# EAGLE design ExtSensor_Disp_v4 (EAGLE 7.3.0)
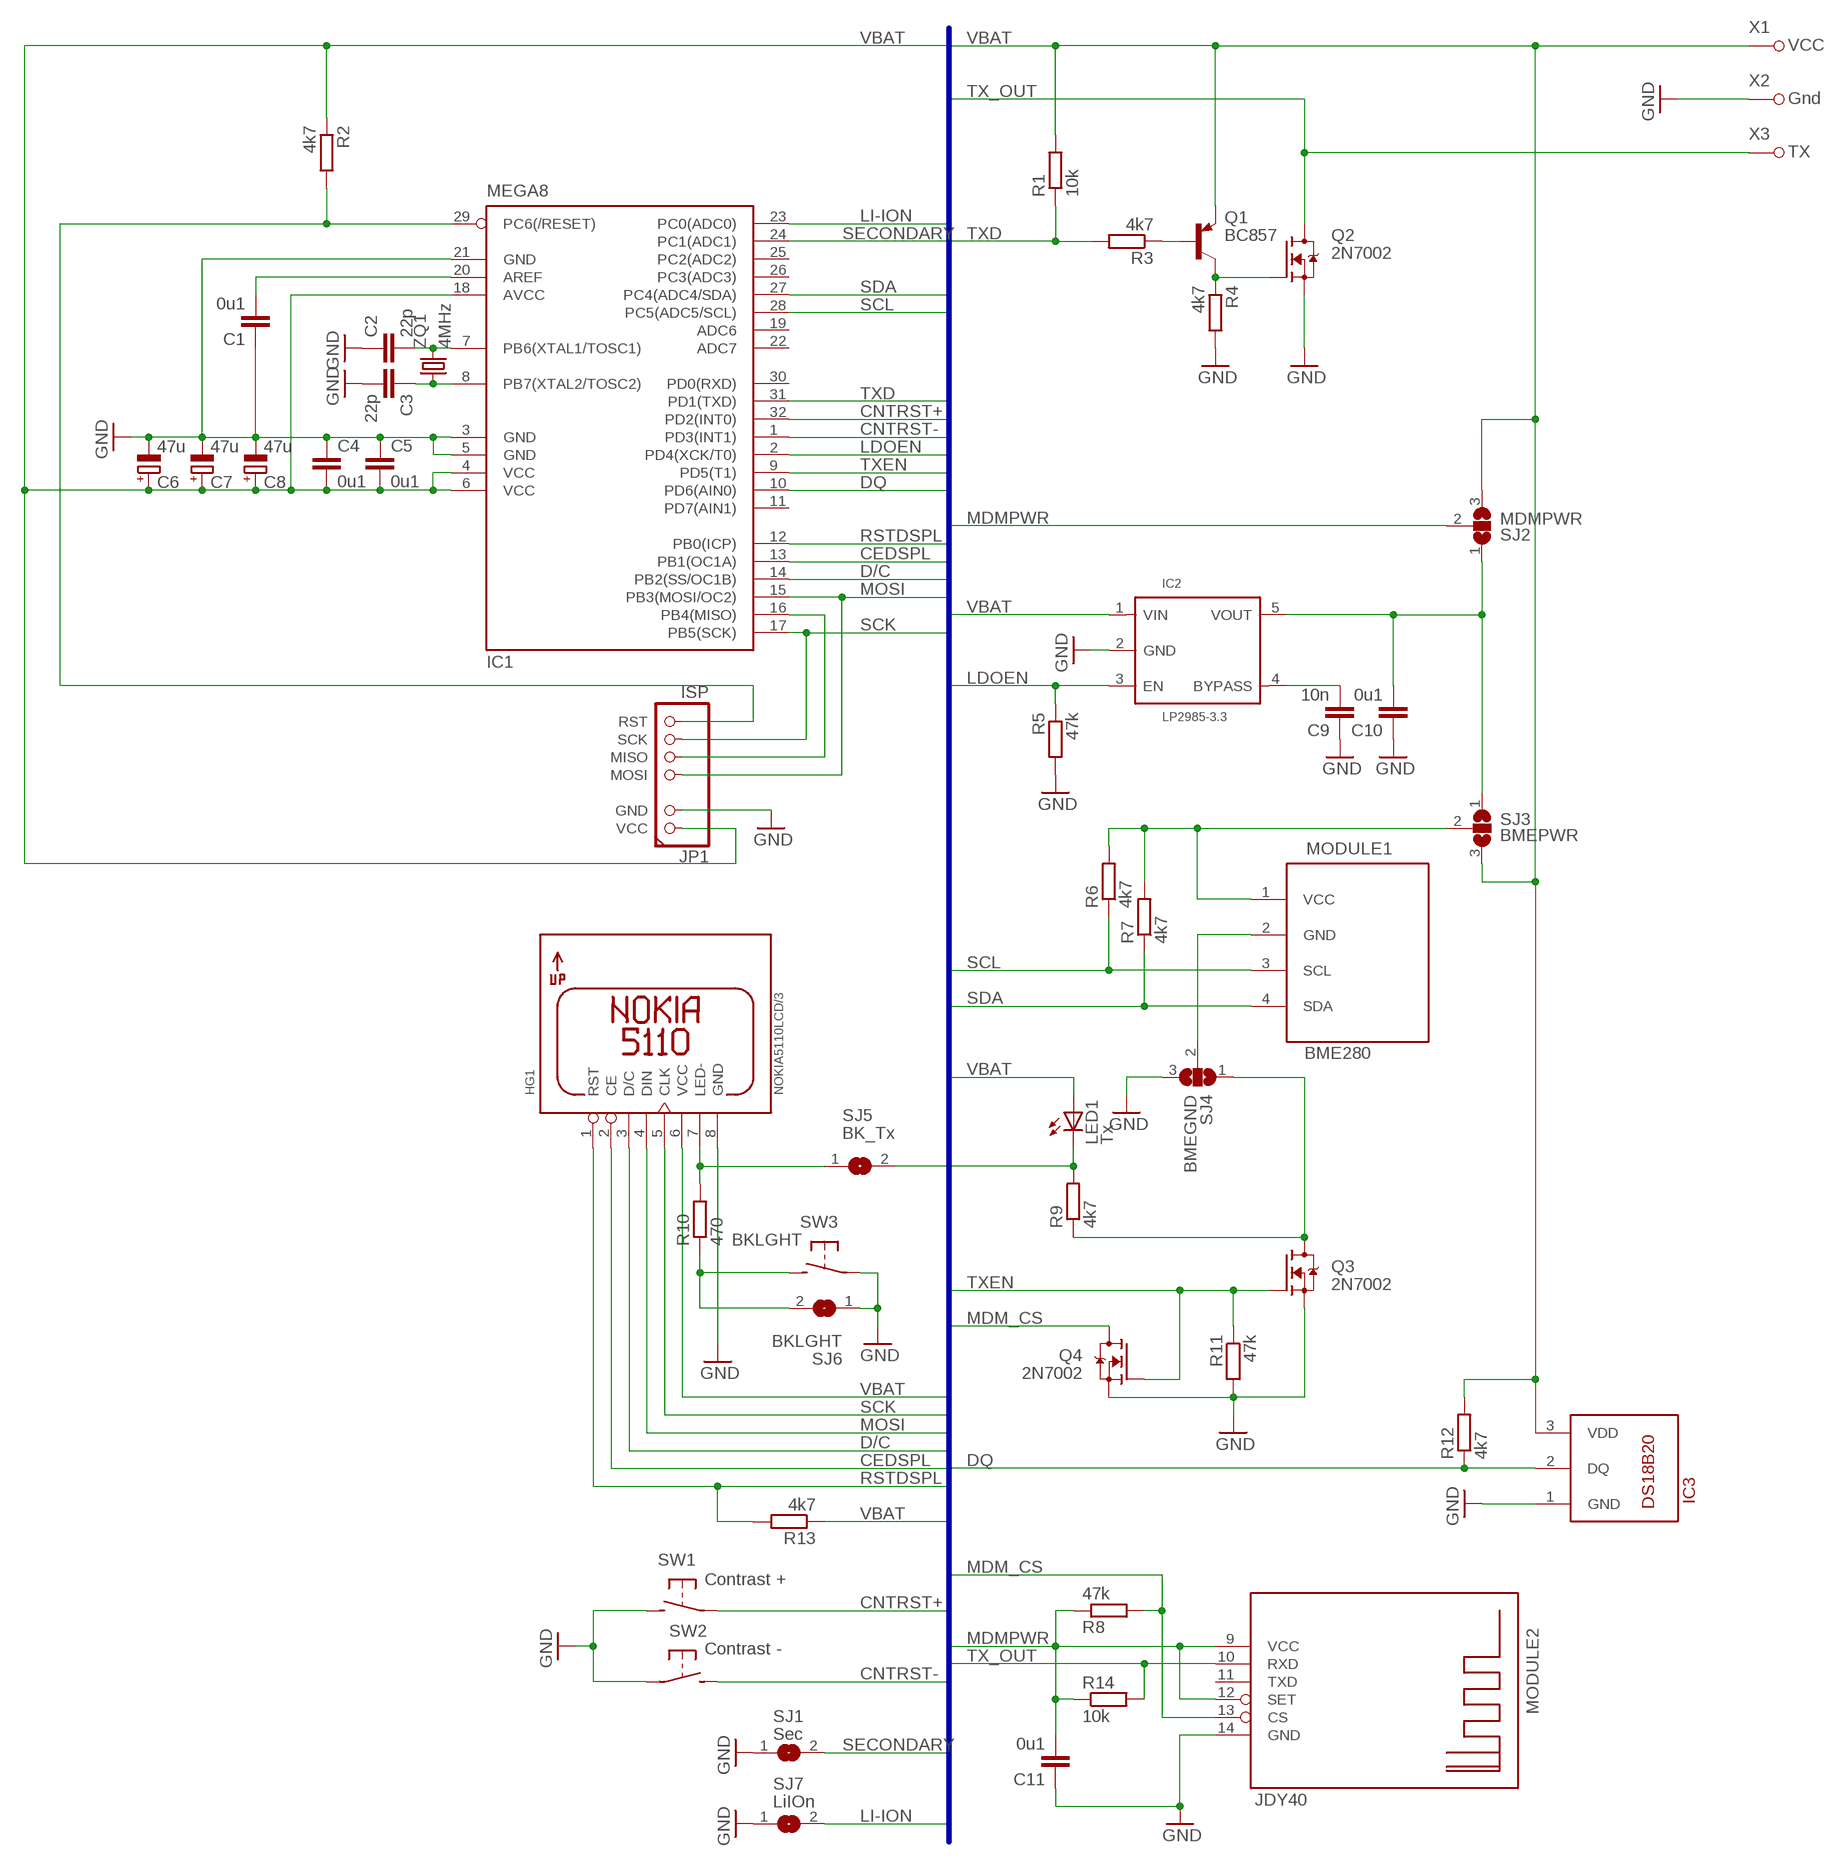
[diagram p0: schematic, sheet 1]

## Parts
C1  0u1  C-EUC0805T  [C0805T]
C2  22p  C-EUC0805T  [C0805T]
C3  22p  C-EUC0805T  [C0805T]
C4  0u1  C-EUC0805T  [C0805T]
C5  0u1  C-EUC0805T  [C0805T]
C6  47u  CPOL-EUE2.5-6  [E2,5-6]
C7  47u  CPOL-EUSMCB  [SMC_B]
C8  47u  CPOL-EUSMCB  [SMC_B]
C9  10n  C-EUC0805T  [C0805T]
C10  0u1  C-EUC0805T  [C0805T]
C11  0u1  C-EUC0805T  [C0805T]
HG1  NOKIA5110LCD/3  [NOKIA5110LCD_V3_NOSILK]
IC1  MEGA8  MEGA8-AI  [TQFP32-08]
IC2  LP2985-3.3  LP2985-XX  [SOT23-5]
IC3  DS18B20  DS18B20/-BH  [TO92-/BIG_HOLES]
JP1  ISP  CONN1X7(2+4)_ISP+/P/NI  [1X07_ISP+POINTS_NO_INF]
LED1  Tx  LED3MM  [LED3MM]
MODULE1  BME280  BM(P|E)280_I2C/4  [BM(P|E)280_I2C_5V]
MODULE2  JDY40  JDY40_NO_GPIO/SMD  [JDY40_NG_SMD]
Q1  BC857  BC857THIN  [SOT23_THIN]
Q2  2N7002  2N7002/THIN  [SOT23_THIN]
Q3  2N7002  2N7002/THIN  [SOT23_THIN]
Q4  2N7002  2N7002/THIN  [SOT23_THIN]
R1  10k  R-EU_R0805T  [R0805T]
R2  4k7  R-EU_R0805T  [R0805T]
R3  4k7  R-EU_R0805T  [R0805T]
R4  4k7  R-EU_R0805T  [R0805T]
R5  47k  R-EU_R0805T  [R0805T]
R6  4k7  R-EU_R0805T  [R0805T]
R7  4k7  R-EU_R0805T  [R0805T]
R8  47k  R-EU_R0805T  [R0805T]
R9  4k7  R-EU_R0805T  [R0805T]
R10  470  R-EU_R0805T  [R0805T]
R11  47k  R-EU_R0805T  [R0805T]
R12  4k7  R-EU_R0805T  [R0805T]
R13  4k7  R-EU_R0805T  [R0805T]
R14  10k  R-EU_R0805T  [R0805T]
SJ1  Sec  SJ  [SJ]
SJ2  MDMPWR  SJ2W  [SJ_2]
SJ3  BMEPWR  SJ2W  [SJ_2]
SJ4  BMEGND  SJ2W  [SJ_2]
SJ5  BK_Tx  SJ  [SJ]
SJ6  BKLGHT  SJ  [SJ]
SJ7  LiIOn  SJ  [SJ]
SW1  Contrast +  TACT_BUTTON  [G72]
SW2  Contrast -  TACT_BUTTON  [G72]
SW3  BKLGHT  TACT_BUTTON  [G72]
X1  VCC  SIMPLE_WIRED_HOLE/1.0MM  [SIMPLE_WIRED_HOLE_1.0]
X2  Gnd  SIMPLE_WIRED_HOLE/1.0MM  [SIMPLE_WIRED_HOLE_1.0]
X3  TX  SIMPLE_WIRED_HOLE/1.0MM  [SIMPLE_WIRED_HOLE_1.0]
ZQ1  4MHz  CRYSTAL_AL/TH  [HC49/S]

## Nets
BMEGND: MODULE1.2(GND) SJ4.2
BMEPWR: MODULE1.1(VCC) R6.2 R7.2 SJ3.2
CEDSPL: HG1.2(CE) IC1.13(PB1(OC1A))
CNTRST+: IC1.32(PD2(INT0)) SW1.S1(P)
CNTRST-: IC1.1(PD3(INT1)) SW2.S2(S)
D/C: HG1.3(D/C) IC1.14(PB2(SS/OC1B))
DQ: IC1.10(PD6(AIN0)) IC3.2(DQ) R12.1
GND: C1.1 C2.1 C3.2 C4.1 C5.1 C6.- C7.- C8.- C9.1 C10.1 C11.1 HG1.8(GND) IC1.3(GND) IC1.5(GND) IC1.21(GND) IC2.2(GND) IC3.1(GND) JP1.GND MODULE2.14(GND) Q2.2(S) Q3.2(S) Q4.2(S) R4.2 R5.2 R11.2 SJ1.1 SJ4.3 SJ6.1 SJ7.1 SW1.S2(S) SW2.S1(P) SW3.S1(P) X2.P$1
LDO_OUT: C10.2 IC2.5(VOUT) SJ2.1 SJ3.1
LDOEN: IC1.2(PD4(XCK/T0)) IC2.3(EN) R5.1
LI-ION: IC1.23(PC0(ADC0)) SJ7.2
MDM_CS: MODULE2.13(CS) Q4.3(D) R8.2
MDMPWR: C11.2 MODULE2.9(VCC) MODULE2.12(SET) R8.1 R14.1 SJ2.2
MISO: IC1.16(PB4(MISO)) JP1.MISO
MOSI: HG1.4(DIN) IC1.15(PB3(MOSI/OC2)) JP1.MOSI
N$1: C3.1 IC1.8(PB7(XTAL2/TOSC2)) ZQ1.1
N$2: Q1.3(C) Q2.1(G) R4.1
N$3: C2.2 IC1.7(PB6(XTAL1/TOSC1)) ZQ1.2
N$4: C9.2 IC2.4(BYPASS)
N$5: HG1.7(LED-) R10.2 SJ5.1
N$7: LED1.K(C) R9.2 SJ5.2
N$9: R10.1 SJ6.2 SW3.S2(S)
N$10: C1.2 IC1.20(AREF)
N$12: Q1.1(B) R3.1
N$16: Q3.3(D) R9.1 SJ4.1
RST: IC1.29(PC6(/RESET)) JP1.RST R2.2
RSTDSPL: HG1.1(RST) IC1.12(PB0(ICP)) R13.2
SCK: HG1.5(CLK) IC1.17(PB5(SCK)) JP1.SCK
SCL: IC1.28(PC5(ADC5/SCL)) MODULE1.3(SCL) R6.1
SDA: IC1.27(PC4(ADC4/SDA)) MODULE1.4(SDA) R7.1
SECONDARY: IC1.24(PC1(ADC1)) SJ1.2
TX_OUT: MODULE2.10(RXD) Q2.3(D) R14.2 X3.P$1
TXD: IC1.31(PD1(TXD)) R1.1 R3.2
TXEN: IC1.9(PD5(T1)) Q3.1(G) Q4.1(G) R11.1
VBAT: C4.2 C5.2 C6.+ C7.+ C8.+ HG1.6(VCC) IC1.4(VCC) IC1.6(VCC) IC1.18(AVCC) IC2.1(VIN) IC3.3(VDD) JP1.+5V(VCC) LED1.A Q1.2(E) R1.2 R2.1 R12.2 R13.1 SJ2.3 SJ3.3 X1.P$1
Unconnected: IC1.11(PD7(AIN1)) IC1.19(ADC6) IC1.22(ADC7) IC1.25(PC2(ADC2)) IC1.26(PC3(ADC3)) IC1.30(PD0(RXD)) MODULE2.11(TXD)

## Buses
VBAT,TXD,SCL,SDA,DQ,MOSI,SCK,D/C,CEDSPL,RSTDSPL,LDOEN,CNTRST-,CNTRST+,TXEN,MDM_CS,MDMPWR,TX_OUT,LI-ION,SECONDARY

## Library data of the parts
C1-C5 C9-C11 = rcl:C-EU: CAPACITOR, European symbol
C6-C8 = rcl:CPOL-EU: POLARIZED CAPACITOR, European symbol
HG1 = lcd-AL:NOKIA5110LCD/3
IC1 = atmel:MEGA8: MICROCONTROLLER 8 Kbytes FLASH, 1 kbytes SRAM, 512 bytes EEPROM, USART, 6-channel 10 bit ADC, 2-channel 8 bit ADC Pin compatible with Atmega48, ATMega88, ATMega168 Source: avr.lbr; MPN: ATMEGA8-16AU; OC_FARNELL: 9171371; OC_NEWARK: 73M8863
IC2 = v-reg-AL:LP2985-XX: Texas Instruments LP2985 150-mA Low-noise Low-dropout Regulator With Shutdown
IC3 = misc-active-AL:DS18B20
JP1 = pinhead-AL:CONN1X7(2+4)_ISP+: PIN HEADER
LED1 = led-AL:LED
MODULE1 = modules-external-AL:BM(P|E)280_I2C
MODULE2 = modules-external-AL:JDY40_NO_GPIO
Q1 = transistor-pnp-AL:BC857*: PNP Transistror
Q2-Q4 = transistor-fet-drv-AL:2N7002: Small signal N-Channel MOSFET transistor
R1-R14 = rcl:R-EU_: RESISTOR, European symbol
SJ1 SJ5-SJ7 = jumper:SJ: SMD solder JUMPER
SJ2-SJ4 = jumper:SJ2W: SMD solder JUMPER
SW1-SW3 = switch-misc-AL:TACT_BUTTON
X1-X3 = connectors-AL:SIMPLE_WIRED_HOLE
ZQ1 = crystal:CRYSTAL_AL

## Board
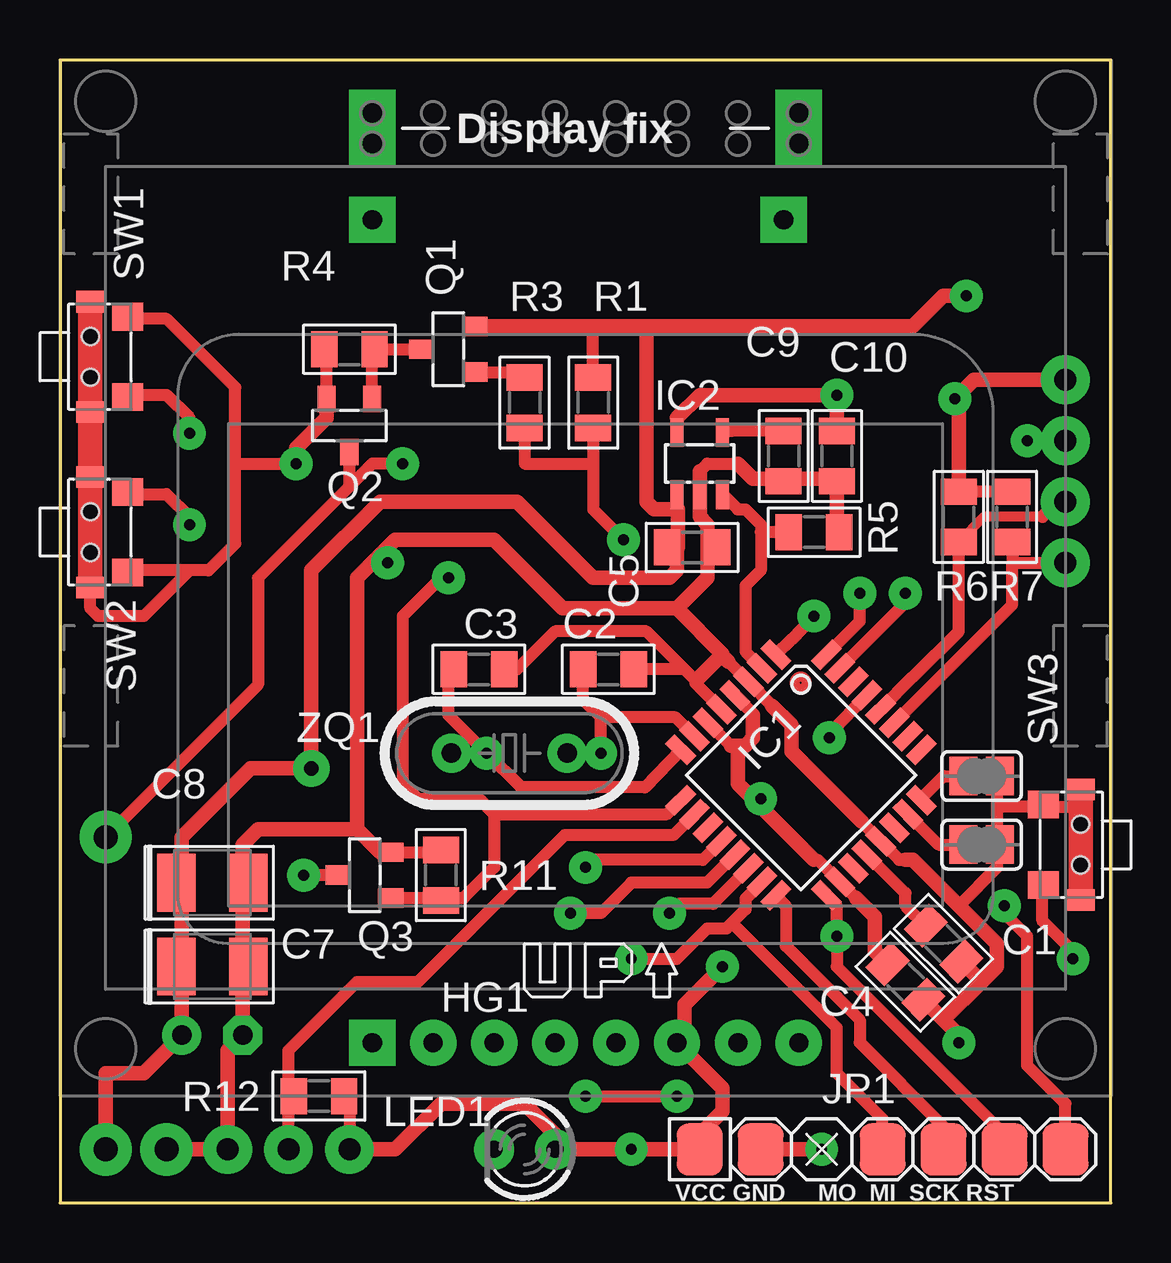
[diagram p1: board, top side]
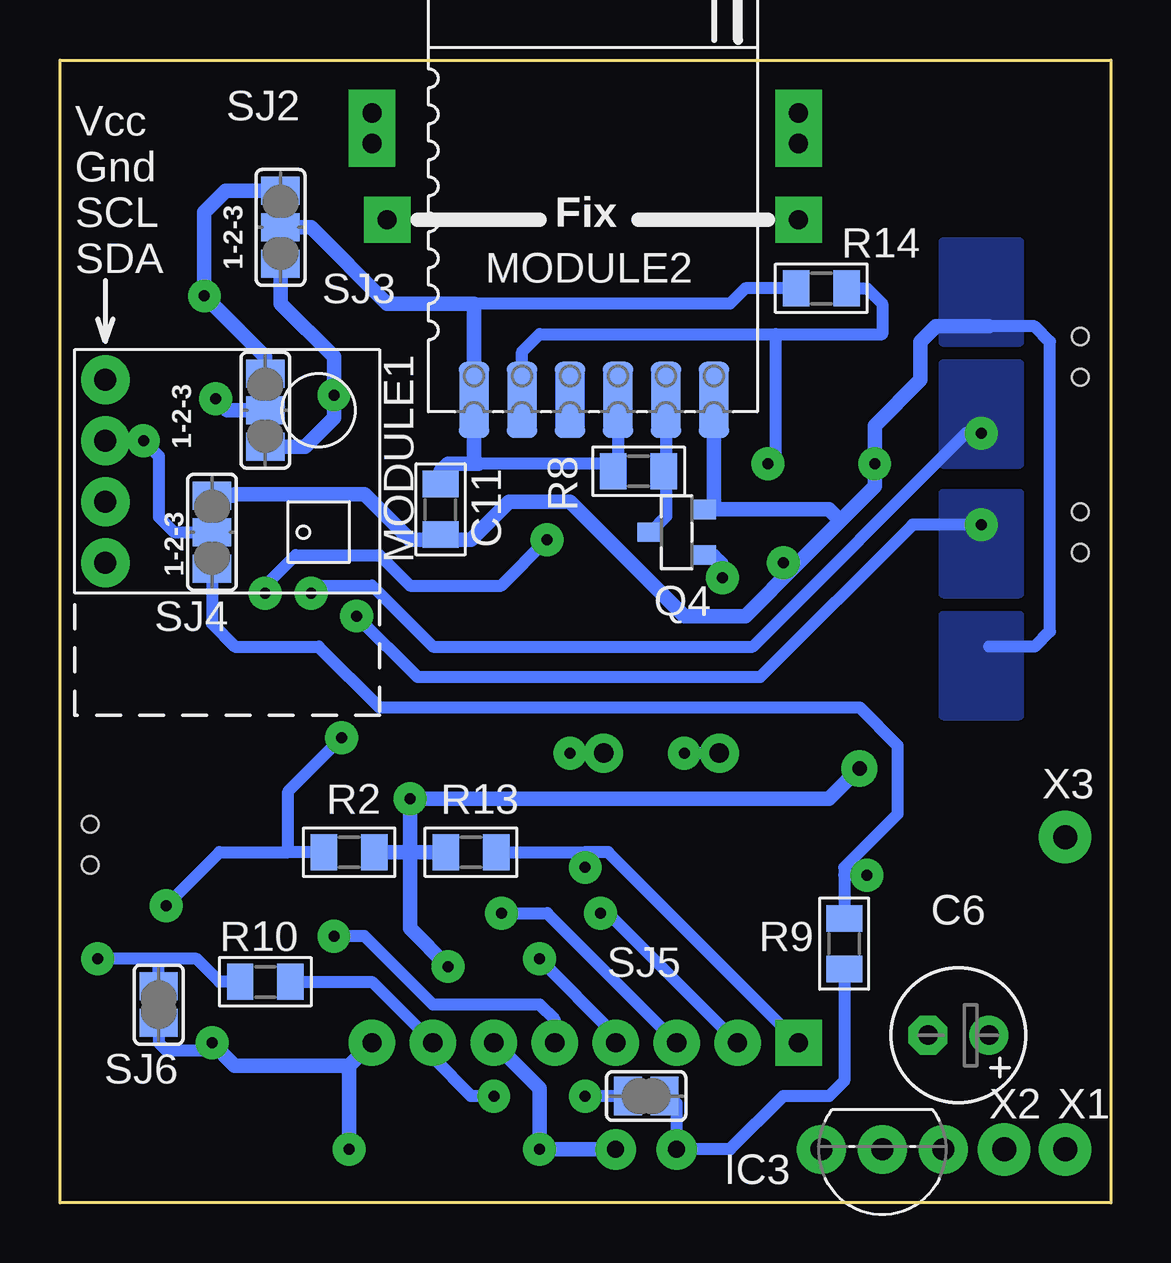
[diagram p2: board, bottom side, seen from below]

Size 43.8 x 47.61 mm. Coordinates in mm from the lower left corner, seen from the top.
Outline: 0,0 43.8,0 43.8,47.61 0,47.61 0,0
Copper layers (1*16): Top 0.035mm / dielectric 1.5mm / Bottom 0.035mm
Design rules "default *": minimum track width 12mil, minimum drill 14mil, track to track 8mil, track to pad 8mil, pad to pad 8mil, via to via 8mil, smd to smd 8mil, copper to edge 20mil, drill to drill 30mil, minimum pad ring 16mil, minimum via ring 18mil, stop-mask expansion 4mil, vias tented up to drill 0mil, thermal gap 8mil

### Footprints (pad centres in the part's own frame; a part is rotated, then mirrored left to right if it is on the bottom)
C0805T = smd 1.1 x 1.5: 1 -1.05,0; 2 1.05,0
E2,5-6 = drill 0.813 pad 1.6: + -1.27,0 | drill 0.813 pad 1.6 octagon: - 1.27,0
SMC_B = smd 1.6 x 2.4: + -1.5,0; - 1.5,0
NOKIA5110LCD_V3_NOSILK = drill 0.8 pad 1.93 square: 1 -8.89,-19.367 | drill 0.8 pad 1.93: 2 -6.35,-19.367; 3 -3.81,-19.367; 4 -1.27,-19.367; 5 1.27,-19.367; 6 3.81,-19.367; 7 6.35,-19.367; 8 8.89,-19.367
TQFP32-08 = smd 1.27 x 0.559: 1 -4.293,2.8; 2 -4.293,2; 3 -4.293,1.2; 4 -4.293,0.4; 5 -4.293,-0.4; 6 -4.293,-1.2; 7 -4.293,-2; 8 -4.293,-2.8; 17 4.293,-2.8; 18 4.293,-2; 19 4.293,-1.2; 20 4.293,-0.4; 21 4.293,0.4; 22 4.293,1.2; 23 4.293,2; 24 4.293,2.8 | smd 0.559 x 1.27: 9 -2.8,-4.293; 10 -2,-4.293; 11 -1.2,-4.293; 12 -0.4,-4.293; 13 0.4,-4.293; 14 1.2,-4.293; 15 2,-4.293; 16 2.8,-4.293; 25 2.8,4.293; 26 2,4.293; 27 1.2,4.293; 28 0.4,4.293; 29 -0.4,4.293; 30 -1.2,4.293; 31 -2,4.293; 32 -2.8,4.293
SOT23-5 = smd 0.55 x 1.2: 1 -0.95,-1.3; 2 0,-1.3; 3 0.95,-1.3; 4 0.95,1.3; 5 -0.95,1.3
TO92-/BIG_HOLES = drill 0.914 pad 2.032: 1 -2.54,0; 2 0,0; 3 2.54,0
1X07_ISP+POINTS_NO_INF = smd 1.905 x 2.159: +5V -7.62,0; GND -5.08,0; MISO 2.54,0; MOSI 0,0; RST 7.62,0; SCK 5.08,0
LED3MM = drill 0.711 pad 1.676: A -1.27,0; K 1.27,0
BM(P|E)280_I2C_5V = drill 0.914 pad 2.032: 1 3.81,5.08; 2 1.27,5.08; 3 -1.27,5.08; 4 -3.81,5.08
JDY40_NG_SMD = smd 1.27 x 3.175: 9 -4.95,-11; 10 -2.95,-11; 11 -0.95,-11; 12 1.05,-11; 13 3.05,-11; 14 5.05,-11
SOT23_THIN = smd 0.8 x 1.1: 1 -0.95,-1.1; 2 0.95,-1.1; 3 0,1.1
R0805T = smd 1.1 x 1.5: 1 -1.05,0; 2 1.05,0
SJ = smd 1.168 x 1.6: 1 -0.762,0; 2 0.762,0
SJ_2 = smd 1.168 x 1.6: 1 -1.524,0; 2 0,0; 3 1.524,0
G72 = smd 0.9 x 1.2: M@0 -2.3,0; M@1 2.3,0 | smd 1.15 x 1.3: S1 -1.675,-1.55; S2 1.675,-1.55 | hole 0.7: -0.85,0; 0.85,0
SIMPLE_WIRED_HOLE_1.0 = drill 1 pad 2.184: P$1 0,0
HC49/S = drill 0.813: 1 -2.413,0; 2 2.413,0

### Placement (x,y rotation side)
C1  36.83,10.79 135 top
C2  22.86,22.23 180 top
C3  17.46,22.23 0 top
C4  35.24,9.21 135 top
C5  26.35,27.3 180 top
C6  6.35,6.99 180 bottom
C7  6.35,9.84 0 top
C8  6.35,13.33 0 top
C9  30.16,31.11 90 top
C10  32.39,31.11 90 top
C11  27.94,28.89 90 bottom
HG1  21.91,26.03 0 top
IC1  30.89,17.82 315 top
IC2  26.67,30.8 0 top
IC3  9.53,2.22 180 bottom
JP1  34.29,2.22 0 top
LED1  19.37,2.22 180 top
MODULE1  36.83,30.48 90 bottom
MODULE2  21.59,44.45 0 bottom
Q1  16.19,35.56 90 top
Q2  12.07,32.38 180 top
Q3  12.7,13.65 90 top
Q4  18.1,27.94 90 bottom
R1  22.23,33.34 90 top
R2  31.75,14.6 180 bottom
R3  19.37,33.34 270 top
R4  12.07,35.56 180 top
R5  31.43,27.94 0 top
R6  37.47,28.57 90 top
R7  39.69,28.57 90 top
R8  19.69,30.48 0 bottom
R9  11.11,10.79 270 bottom
R10  35.24,9.21 0 bottom
R11  15.88,13.65 90 top
R12  10.8,4.45 0 top
R13  26.67,14.6 0 bottom
R14  12.07,38.1 0 bottom
SJ1  38.42,17.78 180 top
SJ2  34.61,40.64 90 bottom
SJ3  35.24,33.02 90 bottom
SJ4  37.47,27.94 90 bottom
SJ5  19.37,4.45 0 bottom
SJ6  39.69,8.26 90 bottom
SJ7  38.42,14.92 180 top
SW1  1.27,35.24 90 top
SW2  1.27,27.94 90 top
SW3  42.55,14.92 270 top
X1  1.91,2.22 0 bottom
X2  4.45,2.22 0 bottom
X3  1.91,15.24 0 bottom
ZQ1  18.73,18.73 0 top

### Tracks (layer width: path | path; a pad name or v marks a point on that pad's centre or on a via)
BMEGND  (via drill 0.46)
  Top 0.508: MODULE1.2 v40.32,31.75
  Bottom 0.508: v40.32,31.75 39.69,31.11 39.69,28.57 39.05,27.94 SJ4.2
BMEPWR  (via drill 0.46)
  Top 0.508: R7.2 R6.2
  Top 0.61: MODULE1.1 38.1,34.29 v37.31,33.5 37.47,33.34 R6.2
  Bottom 0.61: SJ3.2 36.83,33.02 v37.31,33.5
CEDSPL  (via drill 0.46)
  Top 0.508: IC1.13 26.97,13.33 23.81,13.33 22.54,12.06 v21.27,12.06
  Bottom 0.508: v21.27,12.06 20.96,12.06 HG1.2
CNTRST+  (via drill 0.46)
  Top 0.508: v5.4,32.07 5.4,32.7 4.44,33.66 2.91,33.66 SW1.S1 | IC1.32 33.34,24.23 v33.34,25.4
  Bottom 0.508: v33.34,25.4 33.02,25.72 30.8,25.72 28.26,23.18 14.92,23.18 6.03,32.07 v5.4,32.07
  pour Bottom: 6.99,30.8 3.81,30.8 3.81,34.92 6.99,34.92
CNTRST-  (via drill 0.46)
  Top 0.508: v31.43,24.45 30.48,23.46 IC1.1 | 3.18,29.61 3.18,29.53 | 3.18,29.53 4.44,29.53 5.4,28.57 v5.4,28.26 | SW2.S2 2.91,29.53 3.18,29.53
  Bottom 0.508: v31.43,24.45 28.89,21.91 14.61,21.91 8.25,28.26 v5.4,28.26
  pour Bottom: 6.99,25.4 3.81,25.4 3.81,29.53 6.99,29.53
D/C  (via drill 0.46)
  Top 0.508: IC1.14 27.23,12.46 25.79,12.46 v25.4,12.06
  Bottom 0.508: v25.4,12.06 23.5,12.06 HG1.3
DQ
  Top 0.508: IC3.2 9.53,4.45 | 9.53,4.45 9.53,6.35 12.38,9.21 14.92,9.21 21.03,15.32 25.56,15.32 IC1.10 | R12.1 9.53,4.45
GND  (via drill 0.46)
  Top 0.508: 26.67,30.48 26.99,30.8 28.26,30.8 | 32.29,30.16 C10.1 | 32.39,28.04 R5.2 | 13.97,14.6 15.78,14.6 R11.2 | 26.04,22.23 26.35,21.91 26.59,21.83 26.47,21.67 IC1.5 | 29.68,20.71 IC1.3 27.86,22.54 | 7.3,30.8 7.3,27.46 6.19,26.35 5.4,26.35 | 7.3,30.8 7.3,33.97 4.44,36.83 2.91,36.83 SW1.S2 | 5.4,26.35 2.91,26.35 SW2.S1 | 1.27,25.72 1.27,24.77 1.59,24.45 3.49,24.45 5.4,26.35 | 33.42,15.88 33.42,15.86 IC1.21 34.99,14.29 35.24,14.29 | C7.- 7.62,11.43 | 26.04,22.23 C2.1 | 26.04,22.23 24.45,23.81 20.64,23.81 19.05,22.23 C3.2 | 40.91,16.51 SW3.S1 | 40.91,16.51 42.54,16.51 | 7.3,30.8 v9.84,30.8 | Q2.2 11.11,35.46 R4.2 | SJ1.1 39.05,17.78 39.05,16.51 | 39.05,16.51 39.05,14.92 | 39.05,14.92 39.05,13.97 37.47,12.38 | SJ7.1 39.05,14.92 | 40.91,16.51 39.05,16.51
  Top 0.61: v31.75,2.22 JP1.GND | 26.67,30.48 IC2.2 26.67,28.57 26.99,28.26 26.99,27.3 | 28.26,30.8 28.89,30.16 30.16,30.16 | 30.16,30.16 32.29,30.16 | C9.1 30.16,30.16 | 26.99,27.3 26.99,26.03 25.72,24.77 | 7.62,13.33 7.62,11.43 C6.- 6.99,6.35 IC3.1 X2.P$1 | 7.62,13.33 7.62,14.92 8.25,15.56 12.38,15.56 | 25.72,24.77 20.96,24.77 18.1,27.62 13.97,27.62 13.02,26.67 | C5.1 26.99,27.3 | C10.1 32.39,28.04 | 26.59,21.83 27.62,22.86 | 25.72,24.77 27.62,22.86 | Q3.2 13.97,14.6 | 29.68,20.71 30.48,19.91 30.48,18.81 33.42,15.88 | C8.- 7.62,13.33 | 13.97,14.6 13.33,14.6 12.38,15.56 | 35.24,14.29 35.56,14.29 37.47,12.38 39.05,10.79 39.05,9.84 38.42,9.21 | 38.42,9.21 C1.1 | C4.1 36.83,7.62 | 36.83,7.62 | 36.83,7.62 38.42,9.21 | 36.83,7.62 37.47,6.99 v37.47,6.67 | 13.02,26.67 12.38,26.03 12.38,15.56 | v9.84,30.8 9.84,31.43 11.11,32.7 11.11,33.02 Q2.2 | 27.86,22.54 27.62,22.78 27.62,22.86 | 13.02,26.67 v13.65,26.67
  Top 1.016: 1.27,25.72 1.27,37.46 | 42.54,12.7 42.54,16.51 42.54,17.15
  Bottom 0.508: 5.08,36.51 3.18,36.51 2.54,35.88 2.54,23.81 3.18,23.18 5.08,23.18 | SJ6.1 39.69,6.67 39.37,6.35 37.78,6.35 v37.47,6.67
  Bottom 0.61: 31.75,5.72 v31.75,2.22 | HG1.8 31.75,5.72 | 31.75,5.72 36.51,5.72 v37.47,6.67 | SJ4.3 36.58,29.46 36.51,29.53 31.12,29.53 29.21,27.62 27.94,27.62 | 27.94,27.62 26.67,27.62 25.08,29.21 22.54,29.21 17.78,24.45 15.24,24.45 13.02,26.67 | C11.1 27.94,27.62 | 5.08,36.51 7.3,36.51 7.94,35.88 7.94,34.29 9.84,32.38 v9.84,30.8 9.84,29.84 11.27,28.42 | MODULE2.14 16.54,28.92 | 16.54,28.92 16.51,28.89 11.75,28.89 11.27,28.42 | Q4.2 16.57,28.89 16.54,28.92 | 13.02,26.67 11.27,28.42 | v13.65,26.67 13.02,26.67
  pour Bottom: 6.99,35.88 3.81,35.88 3.81,40 6.99,40
  pour Bottom: 6.99,20.32 3.81,20.32 3.81,24.45 6.99,24.45
LDO_OUT  (via drill 0.46)
  Top 0.508: 25.72,32.7 25.72,31.78 IC2.5
  Top 0.61: C10.2 v32.39,33.66 26.67,33.66 25.72,32.7
  Bottom 0.61: SJ3.1 33.59,31.5 32.39,32.7 v32.39,33.66 32.39,35.24 34.61,37.46 SJ2.1
LDOEN
  Top 0.508: IC2.3 27.65,29.5 28.26,28.89 28.57,28.89 29.21,28.26 29.21,27.94 | 29.21,27.94 29.21,26.35 28.57,25.72 28.57,22.96 IC1.2 | R5.1 29.21,27.94
LI-ION
  Top 0.508: IC1.23 36.61,14.92 SJ7.2
MDM_CS
  Bottom 0.508: MODULE2.13 18.54,31.48 18.54,30.57 | 18.54,30.57 R8.2 | 18.54,30.57 18.54,28.6 Q4.3
MDMPWR
  Bottom 0.508: MODULE2.12 20.54,30.89 20.64,30.8 | 20.64,30.8 26.35,30.8 | R14.1 15.24,38.1 15.87,37.46 26.99,37.46 | R8.1 20.74,30.7 20.64,30.8
  Bottom 0.61: 26.54,30.8 MODULE2.9 26.54,37.46 26.99,37.46 30.16,37.46 33.34,40.64 SJ2.2 | C11.2 27.94,30.48 27.62,30.8 26.54,30.8 | 26.54,30.8 26.35,30.8
MISO
  Top 0.508: IC1.16 30.26,12.38 30.26,10.7 33.34,7.62 33.34,6.67 36.83,3.18 JP1.MISO
MOSI  (via drill 0.46)
  Top 0.508: JP1.MOSI 34.29,3.49 32.39,5.4 32.39,7.3 28.02,11.67 | IC1.15 28.57,12.67 28.57,12.22 28.02,11.67 | v23.81,10.16 25.72,10.16 26.99,11.43 27.78,11.43 28.02,11.67
  Bottom 0.508: HG1.4 20.64,6.99 v23.81,10.16
N$1  (via drill 0.46)
  Top 0.508: IC1.8 24.38,17.3 19.21,17.3 v17.78,18.73 16.19,20.32 16.19,22 C3.1
  Bottom 0.508: ZQ1.1 v17.78,18.73
N$2
  Top 0.508: Q2.1 13.01,35.46 R4.1 Q1.3
N$3  (via drill 0.46)
  Top 0.508: IC1.7 25.66,20.22 22.54,20.22 | v22.54,18.73 22.54,20.22 | 22.54,20.22 21.81,20.95 C2.2
  Bottom 0.508: ZQ1.2 v22.54,18.73
N$4
  Top 0.508: C9.2 28,32.16 IC2.4
N$5  (via drill 0.46)
  Top 0.508: v21.91,4.45 v25.72,4.45
  Bottom 0.508: SJ5.1 v21.91,4.45 | v25.72,4.45 26.67,4.45 28.26,6.03 HG1.7 30.8,9.21 R10.2
N$6  (via drill 0.8 pad 1.93)
  other vias: 13.02,40.96
N$7
  Bottom 0.508: R9.2 11.11,5.08 11.75,4.45 13.65,4.45 15.87,2.22 LED1.K 18.1,4.13 18.42,4.45 SJ5.2
N$8  (via drill 0.8 pad 1.93)
  other vias: 30.16,40.96
N$9  (via drill 0.46)
  Top 0.508: v42.23,10.16 42.23,10.48 40.96,11.75 40.96,13.21 SW3.S2
  Bottom 0.508: SJ6.2 39.69,10.16 | R10.1 37.15,9.21 38.1,10.16 39.69,10.16 | 39.69,10.16 v42.23,10.16
N$10
  Top 0.508: IC1.20 35.24,12.9 35.24,12.38 C1.2
N$11  (via drill 0.8 pad 1.93)
  other vias: 13.02,45.4
N$12
  Top 0.508: Q1.1 19.14,34.61 R3.1
N$13  (via drill 0.8 pad 1.93)
  other vias: 13.02,44.13
N$14  (via drill 0.8 pad 1.93)
  other vias: 30.8,45.4
N$15  (via drill 0.8 pad 1.93)
  other vias: 30.8,44.13
N$16  (via drill 0.46)
  Top 0.508: Q3.3 v10.16,13.65
  Bottom 0.508: SJ4.1 37.47,24.13 36.51,23.18 33.02,23.18 30.48,20.64 10.48,20.64 8.89,19.05 8.89,16.19 11.11,13.97 11.11,13.65 | 11.11,13.65 R9.1 | v10.16,13.65 11.11,13.65
RST  (via drill 0.46)
  Top 0.508: IC1.29 32.07,19.56 v32.07,19.37 | JP1.RST 41.91,4.13 40.32,5.72 40.32,11.11 39.37,12.06 v39.37,12.38
  Bottom 0.508: 34.29,14.6 34.29,17.15 v32.07,19.37 | R2.2 34.29,14.6 | v39.37,12.38 37.15,14.6 34.29,14.6
RSTDSPL  (via drill 0.46)
  Top 0.508: IC1.12 26.79,14.29 22.22,14.29 v21.91,13.97
  Bottom 0.508: 13.02,6.35 HG1.1 20.96,14.6 21.91,14.6 | R13.2 21.91,14.6 | v21.91,13.97 21.91,14.6
SCK  (via drill 0.46)
  Top 0.508: JP1.SCK 39.37,2.86 32.39,9.84 v32.39,11.11 32.39,12.36 IC1.17
  Bottom 0.508: HG1.5 23.18,7.62 23.81,8.26 28.26,8.26 31.12,11.11 v32.39,11.11
SCL
  Top 0.406: 40.96,28.57 38.51,28.57 R6.1
  Top 0.508: IC1.28 35.56,21.92 37.47,23.81 R6.1 | MODULE1.3 41.59,29.21 40.96,28.57
SDA
  Top 0.508: R7.1 39.69,26.67 | 39.69,26.67 MODULE1.4 | IC1.27 39.69,24.92 39.69,26.67
SECONDARY
  Top 0.508: IC1.24 35.88,16.79 35.88,16.83 36.83,17.78 SJ1.2
TX_OUT  (via drill 0.46)
  Top 0.508: v14.29,30.8 13.02,30.8 12.07,29.84 | 12.07,29.84 Q2.3 | 12.07,29.84 8.25,26.03 8.25,21.59 X3.P$1
  Bottom 0.508: MODULE2.10 24.54,35.47 23.81,36.2 13.97,36.2 | 13.97,36.2 9.53,36.2 9.53,37.46 10.16,38.1 R14.2 | 13.97,36.2 13.97,31.11 v14.29,30.8
TXD  (via drill 0.46)
  Top 0.508: IC1.31 35.24,25 v35.24,25.4 | 22.22,30.8 19.37,30.8 R3.2 | 22.22,30.8 22.22,28.89 v23.5,27.62 | R1.1 22.22,30.8
  Bottom 0.508: v35.24,25.4 35.24,25.72 33.97,26.99 30.48,26.99 29.21,25.72 25.4,25.72 v23.5,27.62
TXEN  (via drill 0.46)
  Top 0.508: Q3.1 15.87,12.7 | 15.87,12.7 16.83,12.7 18.1,13.97 18.1,16.19 | 18.1,16.19 25.3,16.19 IC1.9 | R11.1 15.87,12.7 | v16.19,26.03 15.87,26.03 14.29,24.45 14.29,17.46 14.92,16.83 17.46,16.83 18.1,16.19
  Bottom 0.508: Q4.1 16.51,26.99 16.19,26.67 v16.19,26.03
VBAT  (via drill 0.46, 0.6)
  Top 0.508: 25.75,28.89 IC2.1 | Q1.2 | IC1.6 27.96,19.05 | IC1.4 28.89,20.38 28.89,20.32 | 33.18,12.7 IC1.18 31.59,14.29 31.43,14.29 | C7.+ 5.08,11.43 | R12.2 12.07,4.45 IC3.3 | R1.2 22.22,36.51
  Top 0.61: 28.26,19.05 28.57,19.05 28.89,19.37 28.89,20.32 | 28.26,19.05 28.26,17.46 29.21,16.51 | v27.62,9.84 26.04,8.26 26.04,6.35 27.62,4.76 27.62,3.81 26.67,2.86 JP1.+5V v23.81,2.22 LED1.A 20.64,2.86 19.37,4.13 15.87,4.13 13.97,2.22 IC3.3 | v29.21,16.83 29.21,16.51 | 24.45,36.51 24.45,29.21 24.76,28.89 25.75,28.89 25.75,27.62 | 25.75,27.62 25.75,27.3 C5.2 | X1.P$1 1.9,5.4 3.49,5.4 C6.+ 5.08,11.43 5.08,13.33 | 5.08,13.33 5.08,15.24 7.94,18.1 v10.48,18.1 10.48,26.35 13.33,29.21 19.05,29.21 22.22,26.03 25.4,26.03 25.72,26.35 25.72,27.59 25.75,27.62 | 24.45,36.51 22.22,36.51 Q1.2 | 24.45,36.51 35.56,36.51 36.83,37.78 v37.78,37.78 | 27.96,19.05 28.26,19.05 | 31.43,14.29 29.21,16.51 | C8.+ 5.08,13.33 | 33.18,12.7 33.97,11.91 33.97,10.48 C4.2
  Bottom 0.61: HG1.6 23.81,4.76 v23.81,2.22 LED1.A | v27.62,9.84 29.21,11.43 29.21,14.6 | 29.21,14.6 v29.21,16.83 11.75,16.83 v10.48,18.1 | R2.1 29.21,14.6 | SJ3.3 35.24,35.24 v37.78,37.78 37.78,41.27 36.89,42.16 SJ2.3 | R13.1 29.21,14.6
(copper drawn outside any net)
  shapes: Top circle x1

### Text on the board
tPlace: Display fix | VCC GND MO MI SCK RST
bPlace: Fix | 1-2-3 | Vcc / Gnd / SCL / SDA | 1-2-3 | 1-2-3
